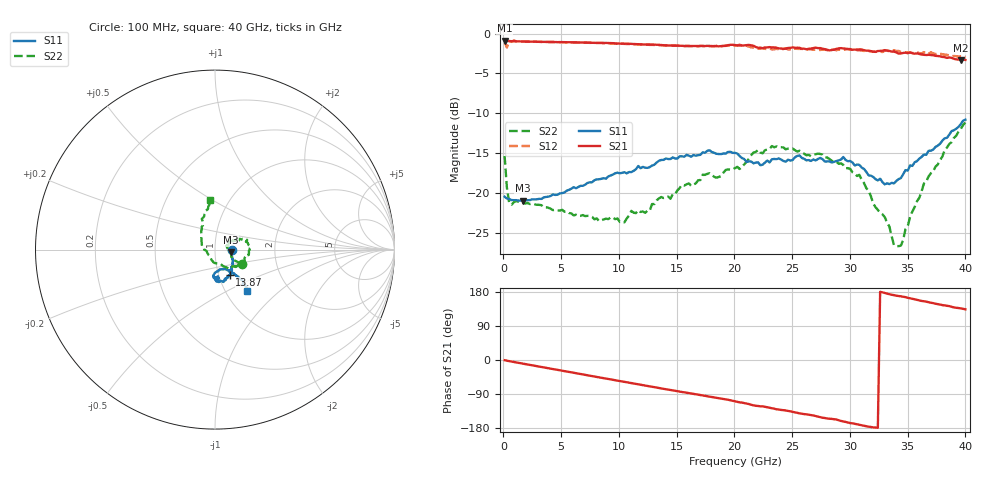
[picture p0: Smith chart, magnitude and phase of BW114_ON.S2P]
!  2-Port S-parameters saved by WinCal
! VAR MeasName=S-Parameters (CALIBRATED_DATA) read from VNA (N5244A)
! VAR MeasDate=9/22/2011 5:00:54 PM
! VAR NAME=L8
! VAR FILENAME=L8.S2P
! VAR DATE=9/22/2011 5:00:54 PM
! VAR PHYS_PORTS=1,2
! VAR ObjTypeName=DATASET
! VAR IndexType=Frequency
# Hz S DB R 50
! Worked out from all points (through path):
!   201 points, 100 MHz to 40 GHz, reference 50 ohm
!   highest |S21| = -0.89 dB at 100 MHz (marker M1); lowest = -3.3 dB at 39.6 GHz (marker M2)
!   group delay of S21, straight-line fit = 15.6 ps
!   lowest |S11| = -20.9 dB at 1.696 GHz (marker M3), VSWR 1.20, Z = 59.7 - j1.69 ohm
!   |S11| at or under -10 dB: start of sweep to end of sweep
!   |S22| runs from -26.6 to -11.2 dB; largest |S21 - S12| = 0.087
!   S11 on the Smith chart (normalised r, x): 100 MHz: 1.21, -0.01; 13.87 GHz: 1.13, -0.32; 40 GHz: 1.26, -0.63
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1e8  -20.43 -2.1  -0.89 -0.6  -1.09 -3.8  -15.34 -28.2
2.995e8  -20.66 -2.0  -0.95 -1.9  -1.74 -4.5  -19.32 -29.7
4.99e8  -20.72 -4.0  -0.94 -3.0  -0.94 -2.6  -21.22 4.7
1.696e9  -20.93 -9.0  -1.00 -9.7  -1.00 -9.7  -21.19 -3.6
6.883e9  -19.07 -28.6  -1.12 -38.1  -1.14 -38.2  -22.73 -0.3
1.0474e10  -17.36 -47.1  -1.28 -57.8  -1.30 -57.9  -23.64 18.2
1.10725e10  -17.35 -47.0  -1.29 -61.3  -1.34 -61.2  -22.21 17.4
1.22695e10  -16.80 -53.4  -1.37 -67.5  -1.40 -67.7  -22.45 25.2
1.34665e10  -15.93 -56.0  -1.42 -74.1  -1.46 -74.0  -20.64 28.7
1.38655e10  -15.82 -59.4  -1.47 -76.2  -1.48 -76.1  -20.60 30.9
1.7257e10  -14.88 -70.8  -1.56 -93.6  -1.56 -94.3  -17.66 24.7
2.005e10  -14.95 -86.7  -1.44 -109.3  -1.49 -109.8  -16.86 24.6
2.22445e10  -16.49 -83.6  -1.77 -122.3  -1.89 -122.2  -14.90 14.0
2.3242e10  -15.75 -83.8  -1.74 -127.4  -1.99 -128.5  -14.09 4.5
2.6833e10  -15.77 -86.4  -1.82 -146.3  -2.03 -147.5  -15.19 -18.1
3.0823e10  -16.45 -92.4  -1.98 -171.0  -2.10 -171.3  -17.69 -54.9
3.34165e10  -18.86 -73.3  -2.18 173.6  -2.22 174.0  -24.15 -107.5
3.38155e10  -18.76 -68.5  -2.26 171.2  -2.10 170.9  -26.47 -123.3
3.4414e10  -18.09 -61.3  -2.49 168.1  -2.31 167.3  -26.55 -169.6
3.6409e10  -15.16 -51.8  -2.67 155.0  -2.33 155.1  -18.78 131.8
3.9601e10  -11.34 -50.0  -3.33 136.3  -2.86 133.1  -11.96 97.0
4e10  -10.79 -52.1  -3.31 133.8  -2.97 130.8  -11.15 95.7
